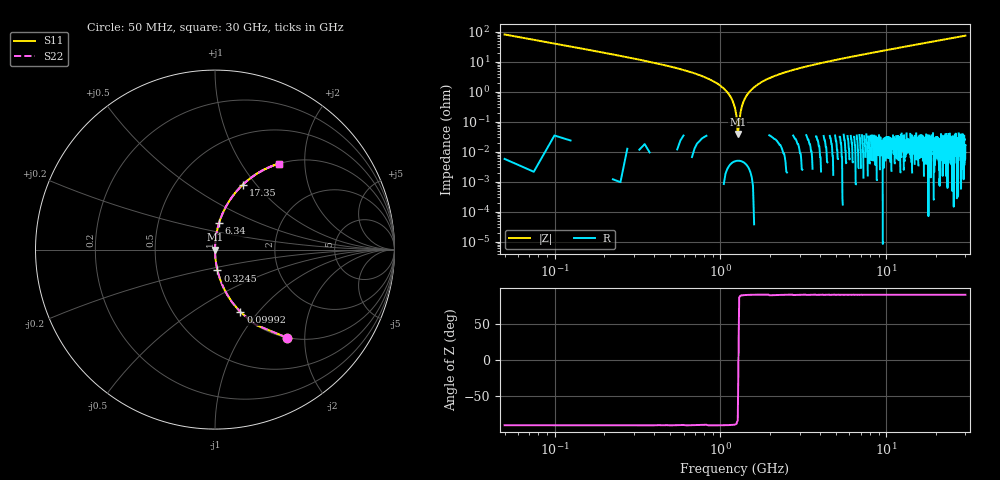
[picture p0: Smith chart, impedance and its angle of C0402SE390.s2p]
!	AVX Thin Film Operation 	Date: April 2014
!	Description: Accu-P® Series, Thin Film  SMD RF Capacitor
!	Part Number: 04023K390FBSTR
# MHZ S MA R 50
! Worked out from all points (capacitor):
!   1201 points, 50 MHz to 30 GHz, reference 50 ohm
!   read as one part in series: C = 39 pF near 199.8 MHz
!   lowest |Z| = 38.8 mohm at 1.273 GHz (marker M1)
!   series resonance near 1.281 GHz, so ESL is about 400 pH
!   S11 on the Smith chart (normalised r, x): 50 MHz: 1.00, -1.63; 99.92 MHz: 1.00, -0.81; 324.5 MHz: 1.00, -0.24; 6.34 GHz: 1.00, +0.30; 17.35 GHz: 1.00, +0.86; 30 GHz: 1.00, +1.49
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50  0.632 -50.8  0.775 39.2  0.775 39.2  0.632 -50.8
99.917  0.376 -67.9  0.926 22.1  0.926 22.1  0.376 -67.9
224.708  0.173 -80.0  0.985 10.0  0.985 10.0  0.173 -80.0
324.542  0.117 -83.2  0.993 6.7  0.993 6.7  0.117 -83.2
948.5  0.019 -88.6  1 1.1  1 1.1  0.019 -88.6
1073.292  0.011 -88.8  1 0.6  1 0.6  0.011 -88.8
1173.125  0.005598 -88.7  1 0.3  1 0.3  0.005598 -88.7
1272.958  0.0003981 -75.4  1 0.0  1 0.0  0.0003981 -75.4
1372.792  0.004431 88.5  1 -0.3  1 -0.3  0.004431 88.5
1497.583  0.01 88.9  1 -0.6  1 -0.6  0.01 88.9
1647.333  0.016 88.7  1 -0.9  1 -0.9  0.016 88.7
1871.958  0.025 88.3  1 -1.4  1 -1.4  0.025 88.3
2196.417  0.036 87.8  0.999 -2.1  0.999 -2.1  0.036 87.8
3294.583  0.069 85.9  0.997 -4.0  0.997 -4.0  0.069 85.9
5041.667  0.117 83.3  0.993 -6.7  0.993 -6.7  0.117 83.3
6339.5  0.15 81.4  0.989 -8.6  0.989 -8.6  0.15 81.4
10058.29  0.239 76.1  0.971 -13.8  0.971 -13.8  0.239 76.1
15025  0.348 69.6  0.937 -20.4  0.937 -20.4  0.348 69.6
17346.12  0.394 66.8  0.919 -23.2  0.919 -23.2  0.394 66.8
20016.67  0.444 63.6  0.896 -26.4  0.896 -26.4  0.444 63.6
25033.29  0.528 58.1  0.849 -31.8  0.849 -31.8  0.528 58.1
30000  0.597 53.3  0.802 -36.7  0.802 -36.7  0.597 53.3
